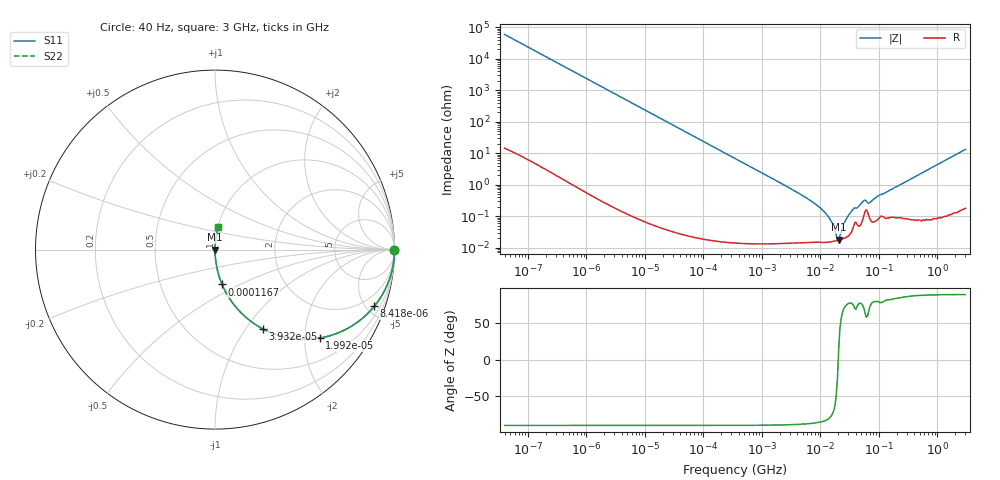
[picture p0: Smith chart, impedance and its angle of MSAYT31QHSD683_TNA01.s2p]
! MSAYT31QHSD683_TNA01  S-PARAMETER MODEL  ( General Type )
! Model Generated by TAIYO YUDEN Corporation (http://www.ty-top.com)
! Version 2.0
! TAIYO YUDEN Control No. 031016
! Copyright(c) 2003 TAIYO YUDEN CO.,LTD. All Rights Reserved.
! Product Description (link to TY-COMPAS)
! https://ds.yuden.co.jp/TYCOMPAS/or/detail?pn=MSAYT31QHSD683KTNA01&u=M
! Products Name : Multilayer Ceramic Capacitors
! Characteristics :
!  Capacitance : 0.068 uF , Rated Voltage : 25V
!  Case Size : 3.2 x 1.6 / 0.126 x 0.063 [mm/inch] , Thickness : 1.15 / 0.045 [mm/inch]
!  (Conditions: Temperature = 25 degC , DC Bias Current/Voltage = 0A / 0V)
! External Node Assignments :
!  1  o---| |---o  2
! GND o---------o GND
! Frequency Range : 40Hz  -  3GHz  [ 401 STEP ]
# MHz S RI R 50
! Freq[MHz].  S11 Real  S11 Imag  S21 Real  S21 Imag  S12 Real  S12 Imag  S22 Real  S22 Imag
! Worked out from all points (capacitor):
!   401 points, 40 Hz to 3 GHz, reference 50 ohm
!   read as one part in series: C = 67.4 nF near 44 Hz
!   lowest |Z| = 17.7 mohm at 20.49 MHz (marker M1)
!   series resonance near 20.16 MHz, so ESL is about 920 pH
!   S11 on the Smith chart (normalised r, x): 40 Hz: open; 8.418 kHz: 1.00, -5.61; 19.92 kHz: 1.00, -2.37; 39.32 kHz: 1.00, -1.20; 116.7 kHz: 1.00, -0.40; 3 GHz: 1.00, +0.26
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4e-05  1 -0.00169  3.28e-06 0.00169  3.28e-06 0.00169  1 -0.00169
0.000834  0.9987 -0.0353  0.00126 0.0353  0.00126 0.0353  0.9987 -0.0353
0.002967  0.9844 -0.1237  0.0156 0.1237  0.0156 0.1237  0.9844 -0.1237
0.008418  0.8871 -0.3163  0.1129 0.3163  0.1129 0.3163  0.8871 -0.3163
0.017386  0.6482 -0.4774  0.3518 0.4774  0.3518 0.4774  0.6482 -0.4774
0.019919  0.584 -0.4927  0.416 0.4927  0.416 0.4927  0.584 -0.4927
0.039317  0.265 -0.4411  0.735 0.4411  0.735 0.4411  0.265 -0.4411
0.064736  0.1175 -0.3217  0.8825 0.3217  0.8825 0.3217  0.1175 -0.3217
0.116704  0.0394 -0.1942  0.9606 0.1942  0.9606 0.1942  0.0394 -0.1942
0.362475  0.00436 -0.0648  0.9956 0.0648  0.9956 0.0648  0.00436 -0.0648
7.222098  0.000154 -0.00285  0.9998 0.00285  0.9998 0.00285  0.000154 -0.00285
13.01976  0.000148 -0.00106  0.9999 0.00106  0.9999 0.00106  0.000148 -0.00106
15.60822  0.000154 -0.000615  0.9998 0.000615  0.9998 0.000615  0.000154 -0.000615
18.71131  0.000165 -0.000174  0.9998 0.000174  0.9998 0.000174  0.000165 -0.000174
20.48705  0.000172 4.27e-05  0.9998 -4.27e-05  0.9998 -4.27e-05  0.000172 4.27e-05
26.8909  0.000207 0.000706  0.9998 -0.000706  0.9998 -0.000706  0.000207 0.000706
35.29647  0.000388 0.00152  0.9996 -0.00152  0.9996 -0.00152  0.000388 0.00152
55.54024  0.00108 0.00294  0.9989 -0.00294  0.9989 -0.00294  0.00108 0.00294
69.67004  0.000826 0.00254  0.9992 -0.00254  0.9992 -0.00254  0.000826 0.00254
150.5692  0.000924 0.00648  0.9991 -0.00648  0.9991 -0.00648  0.000924 0.00648
923.0862  0.00243 0.04  0.9976 -0.04  0.9976 -0.04  0.00243 0.04
3000  0.0185 0.1282  0.9815 -0.1282  0.9815 -0.1282  0.0185 0.1282
